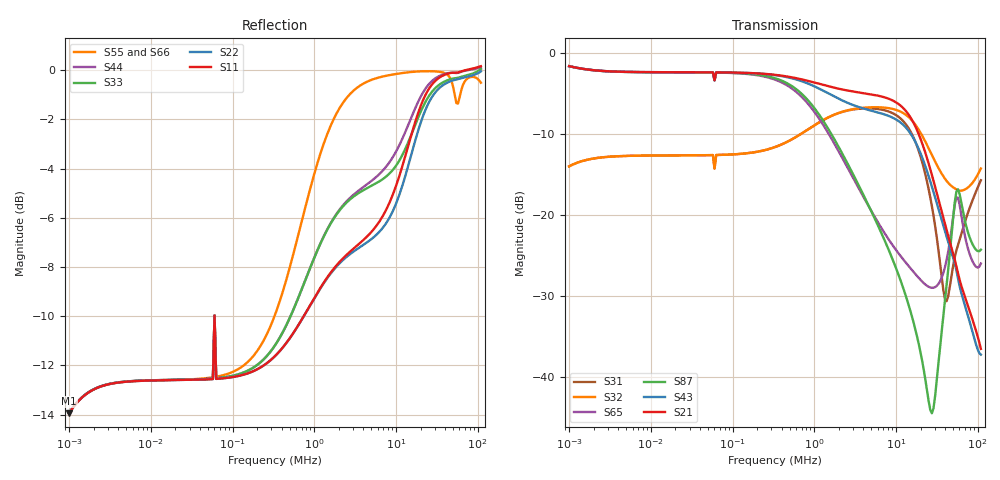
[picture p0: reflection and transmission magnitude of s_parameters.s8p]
! EM Consulting and Software
! Touchstone file was created on 2026-03-05  19:00:33
# HZ S RI R 50.0000
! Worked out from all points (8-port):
!   253 points, 1 kHz to 109.6 MHz, reference 50 ohm
!   strongest paths, dB at 1 kHz, 18.2 kHz, 331.1 kHz, 6.026 MHz, 109.6 MHz:
!     S21: -1.6, -2.3, -2.6, -5.2, -36.5
!     S43: -1.6, -2.3, -2.7, -7.3, -37.2
!     S87: -1.6, -2.3, -3.1, -21.3, -24.2
!     S65: -1.6, -2.3, -3.2, -20.9, -26.0
!     S32: -13.9, -12.6, -11.6, -6.6, -14.2
!     S31: -13.9, -12.6, -11.6, -6.9, -15.7
!   lowest |S11| = -13.9 dB at 1 kHz (marker M1), VSWR 1.50, Z = 68.9 + j14.9 ohm
!   |S11| at or under -10 dB: start of sweep to 60.23 kHz; 60.28 kHz to 742.9 kHz (682.6 kHz wide, 170 % of centre)
